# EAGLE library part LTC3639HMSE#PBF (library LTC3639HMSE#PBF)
High Efficiency, 150V 100mA Synchronous Step-Down Regulator Source: Datasheet
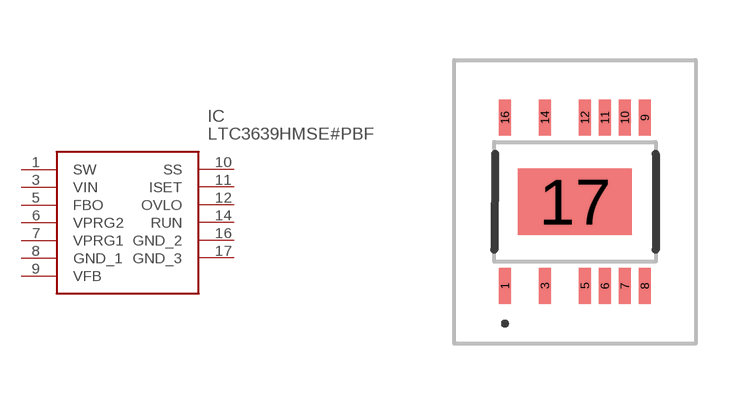
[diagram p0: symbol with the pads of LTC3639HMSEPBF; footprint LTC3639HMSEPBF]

Designator prefix IC

## LTC3639HMSE#PBF (Description: High Efficiency, 150V 100mA Synchronous Step-Down Regulator; Height: 1.1mm; Manufacturer_Name: Analog Devices; Manufacturer_Part_Number: LTC3639HMSE#PBF; Mouser_Part_Number: 584-LTC3639HMSE#PBF; Mouser_Price-Stock: https://www.mouser.co.uk/ProductDetail/Analog-Devices/LTC3639HMSEPBF?qs=hVkxg5c3xu91%2FQQCRu4j6Q%3D%3D)  [LTC3639HMSEPBF]
1  SW
3  VIN
5  FBO
6  VPRG2
7  VPRG1
8  GND_1
9  VFB
10  SS
11  ISET
12  OVLO
14  RUN
16  GND_2
17  GND_3

## Footprint LTC3639HMSEPBF (pad centres in mm)
EXPOSED PAD MINI_SOIC_2023
smd 0.305 x 0.889: 1 -1.75,-2.106; 3 -0.75,-2.106; 5 0.25,-2.106; 6 0.75,-2.106; 7 1.25,-2.106; 8 1.75,-2.106; 9 1.75,2.106; 10 1.25,2.106; 11 0.75,2.106; 12 0.25,2.106; 14 -0.75,2.106; 16 -1.75,2.106
smd 2.845 x 1.651: 17 0,0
